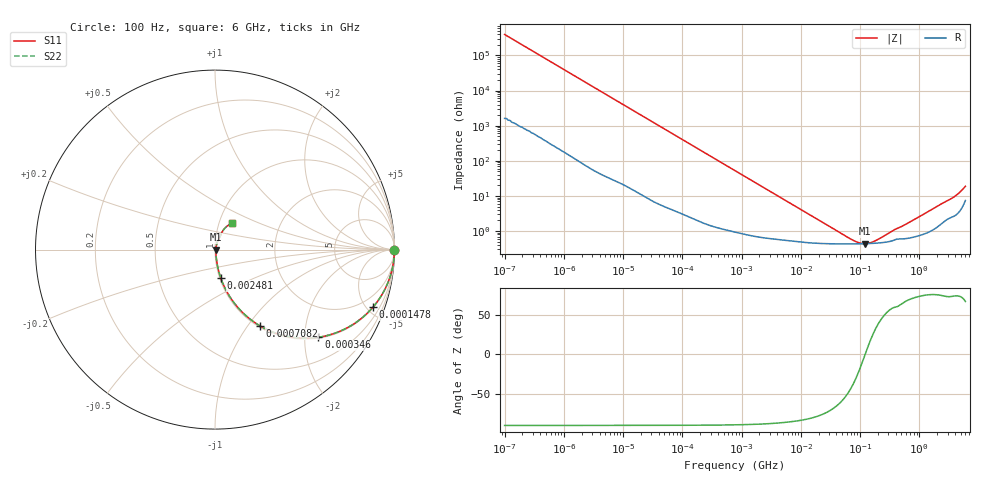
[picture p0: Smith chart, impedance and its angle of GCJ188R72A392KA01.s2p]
!Murata Part Number: GCJ188R72A392KA01
!These Parameters are Measured in Series Mode Connection
!Data Generated on Mar 13, 2026
!  o--ll--o
!Port1  Port2
!  o------o
!Operation Temp=25[degC], DC Bias Voltage=0[V]
!Freq. Start=100[Hz] Stop=6[GHz] 401[Steps]
# Hz S RI R 50
!Freq.(Hz) S11(Real) S11(Imag) S21(Real) S21(Imag) S12(Real) S12(Imag) S22(Real) S22(Imag)
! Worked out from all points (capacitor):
!   401 points, 100 Hz to 6 GHz, reference 50 ohm
!   read as one part in series: C = 4.03 nF near 109 Hz
!   lowest |Z| = 437 mohm at 122 MHz (marker M1)
!   series resonance near 121.9 MHz, so ESL is about 420 pH
!   S11 on the Smith chart (normalised r, x): 100 Hz: open; 147.8 kHz: 1.05, -5.45; 346 kHz: 1.03, -2.34; 708.2 kHz: 1.02, -1.15; 2.481 MHz: 1.01, -0.33; 6 GHz: 1.15, +0.35
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100  1 -0.000254  1.1e-06 0.000254  1.1e-06 0.000254  1 -0.000254
2008  1 -0.00505  4.73e-05 0.00505  4.73e-05 0.00505  1 -0.00505
12592  0.9988 -0.0315  0.00116 0.0315  0.00116 0.0315  0.9988 -0.0315
40335  0.9894 -0.0995  0.0106 0.0995  0.0106 0.0995  0.9894 -0.0995
86348  0.9545 -0.2047  0.0455 0.2047  0.0455 0.2047  0.9545 -0.2047
147774  0.8794 -0.3215  0.1206 0.3215  0.1206 0.3215  0.8794 -0.3215
221108  0.7671 -0.4181  0.2329 0.4181  0.2329 0.4181  0.7671 -0.4181
345986  0.5764 -0.4885  0.4236 0.4885  0.4236 0.4885  0.5764 -0.4885
495019  0.4022 -0.4835  0.5978 0.4835  0.5978 0.4835  0.4022 -0.4835
708247  0.2507 -0.4251  0.7493 0.4251  0.7493 0.4251  0.2507 -0.4251
774597  0.2196 -0.4052  0.7804 0.4052  0.7804 0.4052  0.2196 -0.4052
1325623  0.092 -0.2769  0.908 0.2769  0.908 0.2769  0.092 -0.2769
2481164  0.0323 -0.1585  0.9677 0.1585  0.9677 0.1585  0.0323 -0.1585
5554849  0.0108 -0.0729  0.9892 0.0729  0.9892 0.0729  0.0108 -0.0729
1.555665e7  0.00524 -0.0262  0.9948 0.0262  0.9948 0.0262  0.00524 -0.0262
7.455971e7  0.00431 -0.00349  0.9957 0.00349  0.9957 0.00349  0.00431 -0.00349
9.753859e7  0.00432 -0.00153  0.9957 0.00153  0.9957 0.00153  0.00432 -0.00153
1.220122e8  0.00436 7e-06  0.9956 -7e-06  0.9956 -7e-06  0.00436 7e-06
1.745687e8  0.00448 0.00249  0.9955 -0.00249  0.9955 -0.00249  0.00448 0.00249
3.124326e8  0.00506 0.00732  0.9949 -0.00732  0.9949 -0.00732  0.00506 0.00732
3.505958e9  0.0301 0.0768  0.9699 -0.0768  0.9699 -0.0768  0.0301 0.0768
6e9  0.0926 0.1461  0.9074 -0.1461  0.9074 -0.1461  0.0926 0.1461
